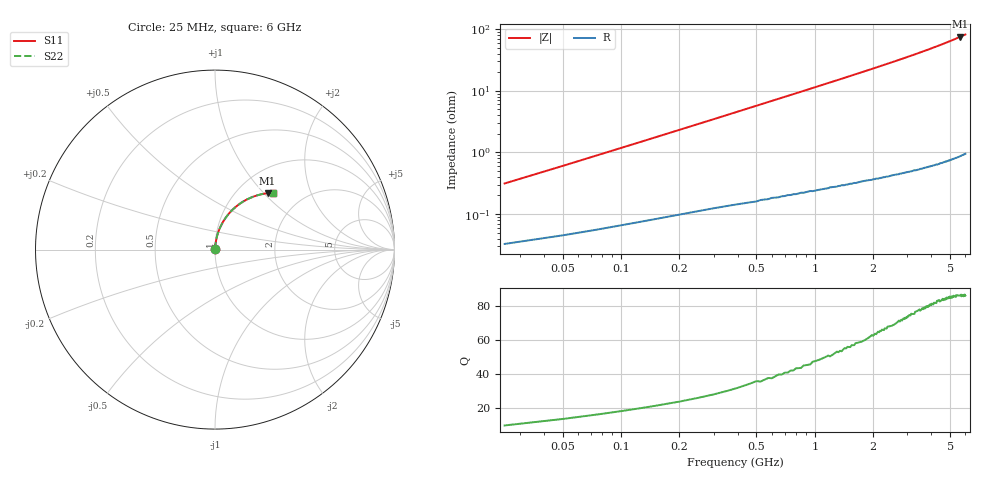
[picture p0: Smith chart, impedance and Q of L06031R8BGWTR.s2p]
!	AVX Thin Film Operation
!	Date:	March	2003
!	Description: Accu-L® Series Thin Film SMD RF Inductors
!	Part Number: L06031R8BGWTR
!	25MHz-6GHz
!	Serial	Measurements
#	mhz	S	db	R	50
!	S11	S11	S21	S21	S12	S12	S22	S22
!	dB	Phase	dB	Phase	dB	Phase	dB	Phase
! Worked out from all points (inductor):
!   240 points, 25 MHz to 6 GHz, reference 50 ohm
!   read as 1/Y11, port 2 shorted: L = 1.89 nH near 50 MHz
!   highest Q = 86.4 at 5.65 GHz (marker M1), where L = 2.12 nH
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25  -52.11 82.5  -0.00 -0.2  -0.00 -0.2  -52.11 82.5
50  -46.47 84.1  -0.00 -0.4  -0.00 -0.4  -46.47 84.1
75  -43.12 84.7  -0.01 -0.6  -0.01 -0.6  -43.12 84.7
100  -40.73 85.0  -0.01 -0.8  -0.01 -0.8  -40.73 85.0
125  -38.86 85.2  -0.01 -1.0  -0.01 -1.0  -38.86 85.2
175  -36.04 85.3  -0.01 -1.4  -0.01 -1.4  -36.04 85.3
225  -33.92 85.2  -0.01 -1.8  -0.01 -1.8  -33.92 85.2
275  -32.23 85.1  -0.01 -2.2  -0.01 -2.2  -32.23 85.1
325  -30.82 84.9  -0.01 -2.6  -0.01 -2.6  -30.82 84.9
400  -29.06 84.5  -0.02 -3.2  -0.02 -3.2  -29.06 84.5
575  -25.98 83.4  -0.03 -4.6  -0.03 -4.6  -25.98 83.4
775  -23.45 82.1  -0.04 -6.2  -0.04 -6.2  -23.45 82.1
1025  -21.07 80.3  -0.06 -8.1  -0.06 -8.1  -21.07 80.3
1250  -19.39 78.7  -0.07 -9.9  -0.07 -9.9  -19.39 78.7
1475  -18.00 77.0  -0.10 -11.6  -0.10 -11.6  -18.00 77.0
2025  -15.35 73.0  -0.16 -15.9  -0.16 -15.9  -15.35 73.0
2475  -13.69 69.7  -0.23 -19.3  -0.23 -19.3  -13.69 69.7
3025  -12.06 65.6  -0.32 -23.5  -0.32 -23.5  -12.06 65.6
4025  -9.82 58.4  -0.52 -30.9  -0.52 -30.9  -9.82 58.4
5025  -8.17 51.3  -0.77 -38.0  -0.77 -38.0  -8.17 51.3
5650  -7.34 47.0  -0.94 -42.4  -0.94 -42.4  -7.34 47.0
6000  -6.93 44.7  -1.04 -44.8  -1.04 -44.8  -6.93 44.7
